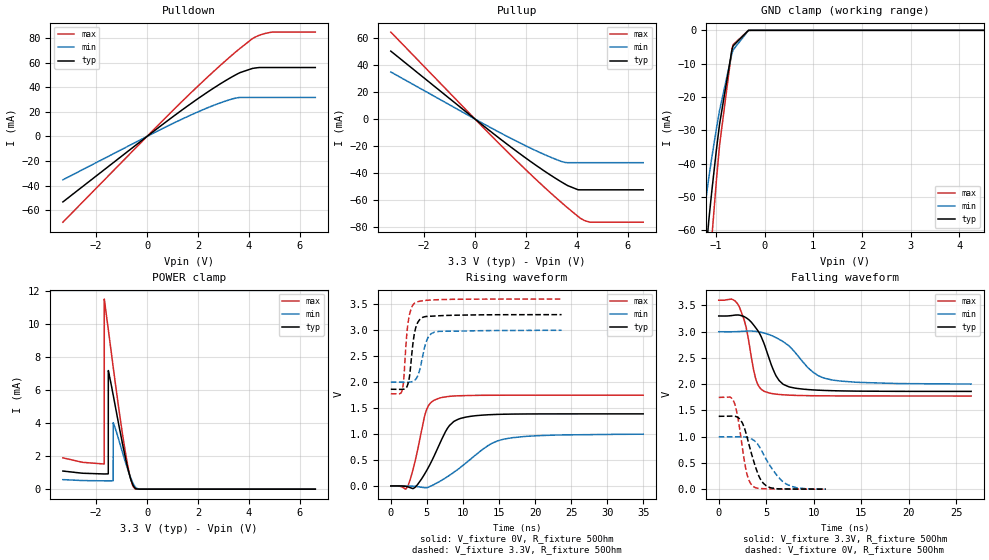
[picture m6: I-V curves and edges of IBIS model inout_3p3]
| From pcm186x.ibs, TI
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|   inout_3p3 Model
[Model]   inout_3p3
Model_type   I/O
Polarity   Non-Inverting
Enable   Active-High
Vinl = 0.99
Vinh = 2.31
Vmeas = 1.65
Vref = 0
Cref = 20pF
Rref = 150
|   typ   min   max
|   (nom PVT)   (fast PVT)   (slow PVT)
C_comp   6.104e-12   5.727e-12   6.322e-12
[Model spec]
|subparameter
Vinl   0.99   0.9   1.08
Vinh   2.31   2.1   2.52
| Where nom  PVT is Nominal Process, 3.3V, 27C
|   Fast PVT is Strong Process,  3.6V, -40C
|   Slow PVT is Weak Process,   3V, 125C
[Voltage Range]   3.3   3   3.6
|Junction Temperature
[Temperature Range]   27   125   -40
[Pullup Reference]   3.3   3   3.6
[Pulldown Reference]   0   0   0
[Power Clamp Reference]   3.3   3   3.6
[GND Clamp Reference]   0   0   0
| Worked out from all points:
|   slope of the pulldown table from 0 to 0.495 V, typ, clamps not added: 62.7 ohm
|   slope of the pullup table from 0 to 0.495 V, typ, clamps not added: 66.6 ohm
|   POWER clamp passes 1 mA (typ) near -0.71 V on its own axis
|   falling waveform, V_fixture 3.3V, R_fixture 50Ohm: 20-80 % time 1.92ns typ, 3.28ns min, 1.18ns max; typ from 3.3 V to 1.86 V
|   rising waveform, V_fixture 0V, R_fixture 50Ohm: 20-80 % time 2.97ns typ, 5.65ns min, 1.65ns max; typ from 0 V to 1.39 V
|   rising waveform, V_fixture 3.3V, R_fixture 50Ohm: 20-80 % time 764ps typ, 1.04ns min, 662ps max; typ from 1.86 V to 3.3 V
|   falling waveform, V_fixture 0V, R_fixture 50Ohm: 20-80 % time 1.36ns typ, 2.11ns min, 914ps max; typ from 1.39 V to 0.001 V
[Pulldown]
|   Voltage   I(typ)   I(min)   I(max)
-3.3V     -53.23mA   -35.26mA   -69.7mA
459mV     7.331mA    4.841mA    9.639mA
2.043V    31.34mA    20.36mA    41.79mA
2.826V    42.1mA     26.91mA    56.8mA
3.392V    49.08mA    30.72mA    67.12mA
3.633V    51.73mA    31.68mA    71.31mA
4.131V    55.24mA    31.68mA    79.38mA
4.402V    55.97mA    31.68mA    82.17mA
4.919V    55.97mA    31.68mA    84.78mA
6.6V      55.97mA    31.68mA    84.78mA
[GND Clamp]
|   Voltage   I(typ)   I(min)   I(max)
-3.3V     -1.542A    -1.263A    -1.822A
-1.373V   -93.75mA   -69.09mA   -125.9mA
-1.14V    -56.29mA   -43.7mA    -73.49mA
-1.086V   -48.56mA   -38.37mA   -62.69mA
-986.7mV  -35.57mA   -29.3mA    -44.65mA
-924mV    -28.14mA   -24.02mA   -34.45mA
-672mV    -6.037mA   -7.11mA    -5.9mA
-646.8mV  -4.683mA   -5.888mA   -4.309mA
-330mV    -4.074uA   -38.34uA   -407.4nA
6.6V      0A         0A         0A
[Pullup]
|   Voltage   I(typ)   I(min)   I(max)
-3.3V     50.26mA    34.82mA    64.35mA
459mV     -6.903mA   -4.78mA    -8.872mA
2.168V    -31.26mA   -21.45mA   -40.7mA
3.456V    -47.31mA   -31.79mA   -62.85mA
4.043V    -52.36mA   -32.34mA   -72.11mA
4.143V    -52.43mA   -32.34mA   -73.55mA
4.287V    -52.43mA   -32.34mA   -75.11mA
4.505V    -52.43mA   -32.34mA   -76.34mA
6.6V      -52.43mA   -32.34mA   -76.38mA
[POWER Clamp]
|   Voltage   I(typ)   I(min)   I(max)
-3.3V     1.099mA    579.3uA    1.9mA
-1.68V    922uA      505.5uA    1.525mA
-1.676V   922uA      505.5uA    11.52mA
-1.521V   925.9uA    504.4uA    9.707mA
-1.518V   7.19mA     504.4uA    9.668mA
-1.329V   5.72mA     512.3uA    7.426mA
-1.326V   5.695mA    4.029mA    7.391mA
-963.6mV  2.762mA    2.233mA    3.353mA
-807mV    1.617mA    1.438mA    1.862mA
-632.4mV  573.7uA    655.1uA    559.7uA
-480mV    75.5uA     171.6uA    38.95uA
6.6V      0A         0A         0A
[Ramp]
R_load = 50
|   typ   min   max
dV/dt_r   0.833088/2.9679e-09   0.598181/5.62505e-09   1.04915/1.65098e-09
dV/dt_f   0.862208/1.91294e-09   0.599473/3.26309e-09   1.09494/1.17996e-09
[Falling Waveform]
V_fixture = 3.3V
V_fixture_min = 3V
V_fixture_max = 3.6V
R_fixture = 50Ohm
|   Time   V(typ)   V(min)   V(max)
0s        3.3V       3V         3.6V
2.11ns    3.318V     3.004V     3.494V
2.9ns     3.264V     3.012V     3.069V
3.86ns    3.083V     3.007V     2.122V
4.81ns    2.753V     2.973V     1.863V
6.02ns    2.162V     2.888V     1.811V
7.46ns    1.947V     2.718V     1.792V
9.9ns     1.892V     2.232V     1.781V
11.96ns   1.877V     2.079V     1.778V
26.54ns   1.863V     2.003V     1.775V
[Rising Waveform]
V_fixture = 0V
V_fixture_min = 0V
V_fixture_max = 0V
R_fixture = 50Ohm
|   Time   V(typ)   V(min)   V(max)
0s        639.6pV    34.49nV    440.6pV
2.21ns    -11.4mV    -122.4uV   -41.59mV
3.31ns    -31.9mV    -6.563mV   445.5mV
4.89ns    278.6mV    -32.92mV   1.444V
6.69ns    787mV      80.3mV     1.69V
7.93ns    1.126V     186.5mV    1.723V
9.14ns    1.272V     303.8mV    1.736V
13.46ns   1.371V     776.5mV    1.747V
15.61ns   1.381V     899.8mV    1.748V
34.98ns   1.388V     997mV      1.749V
[Rising Waveform]
V_fixture = 3.3V
V_fixture_min = 3V
V_fixture_max = 3.6V
R_fixture = 50Ohm
|   Time   V(typ)   V(min)   V(max)
0s        1.863V     2.001V     1.775V
1.54ns    1.861V     2V         1.825V
1.78ns    1.864V     1.999V     2.032V
2.17ns    1.897V     1.998V     2.848V
2.41ns    1.984V     1.998V     3.161V
3.34ns    2.984V     2.037V     3.526V
4.02ns    3.206V     2.243V     3.558V
5.11ns    3.266V     2.848V     3.578V
6.03ns    3.273V     2.962V     3.585V
23.66ns   3.3V       2.999V     3.6V
[Falling Waveform]
V_fixture = 0V
V_fixture_min = 0V
V_fixture_max = 0V
R_fixture = 50Ohm
|   Time   V(typ)   V(min)   V(max)
0s        1.388V     997mV      1.749V
1.17ns    1.391V     996.7mV    1.755V
1.63ns    1.391V     997.8mV    1.651V
2.29ns    1.32V      998.2mV    1.038V
2.93ns    1.026V     987.9mV    316.9mV
3.58ns    591.5mV    943.8mV    58.85mV
4.37ns    195.6mV    779.4mV    12.54mV
5.42ns    28.43mV    439.4mV    5.321mV
7.71ns    3.323mV    50.7mV     1.433mV
11.25ns   971.8uV    2.257mV    481.1uV
